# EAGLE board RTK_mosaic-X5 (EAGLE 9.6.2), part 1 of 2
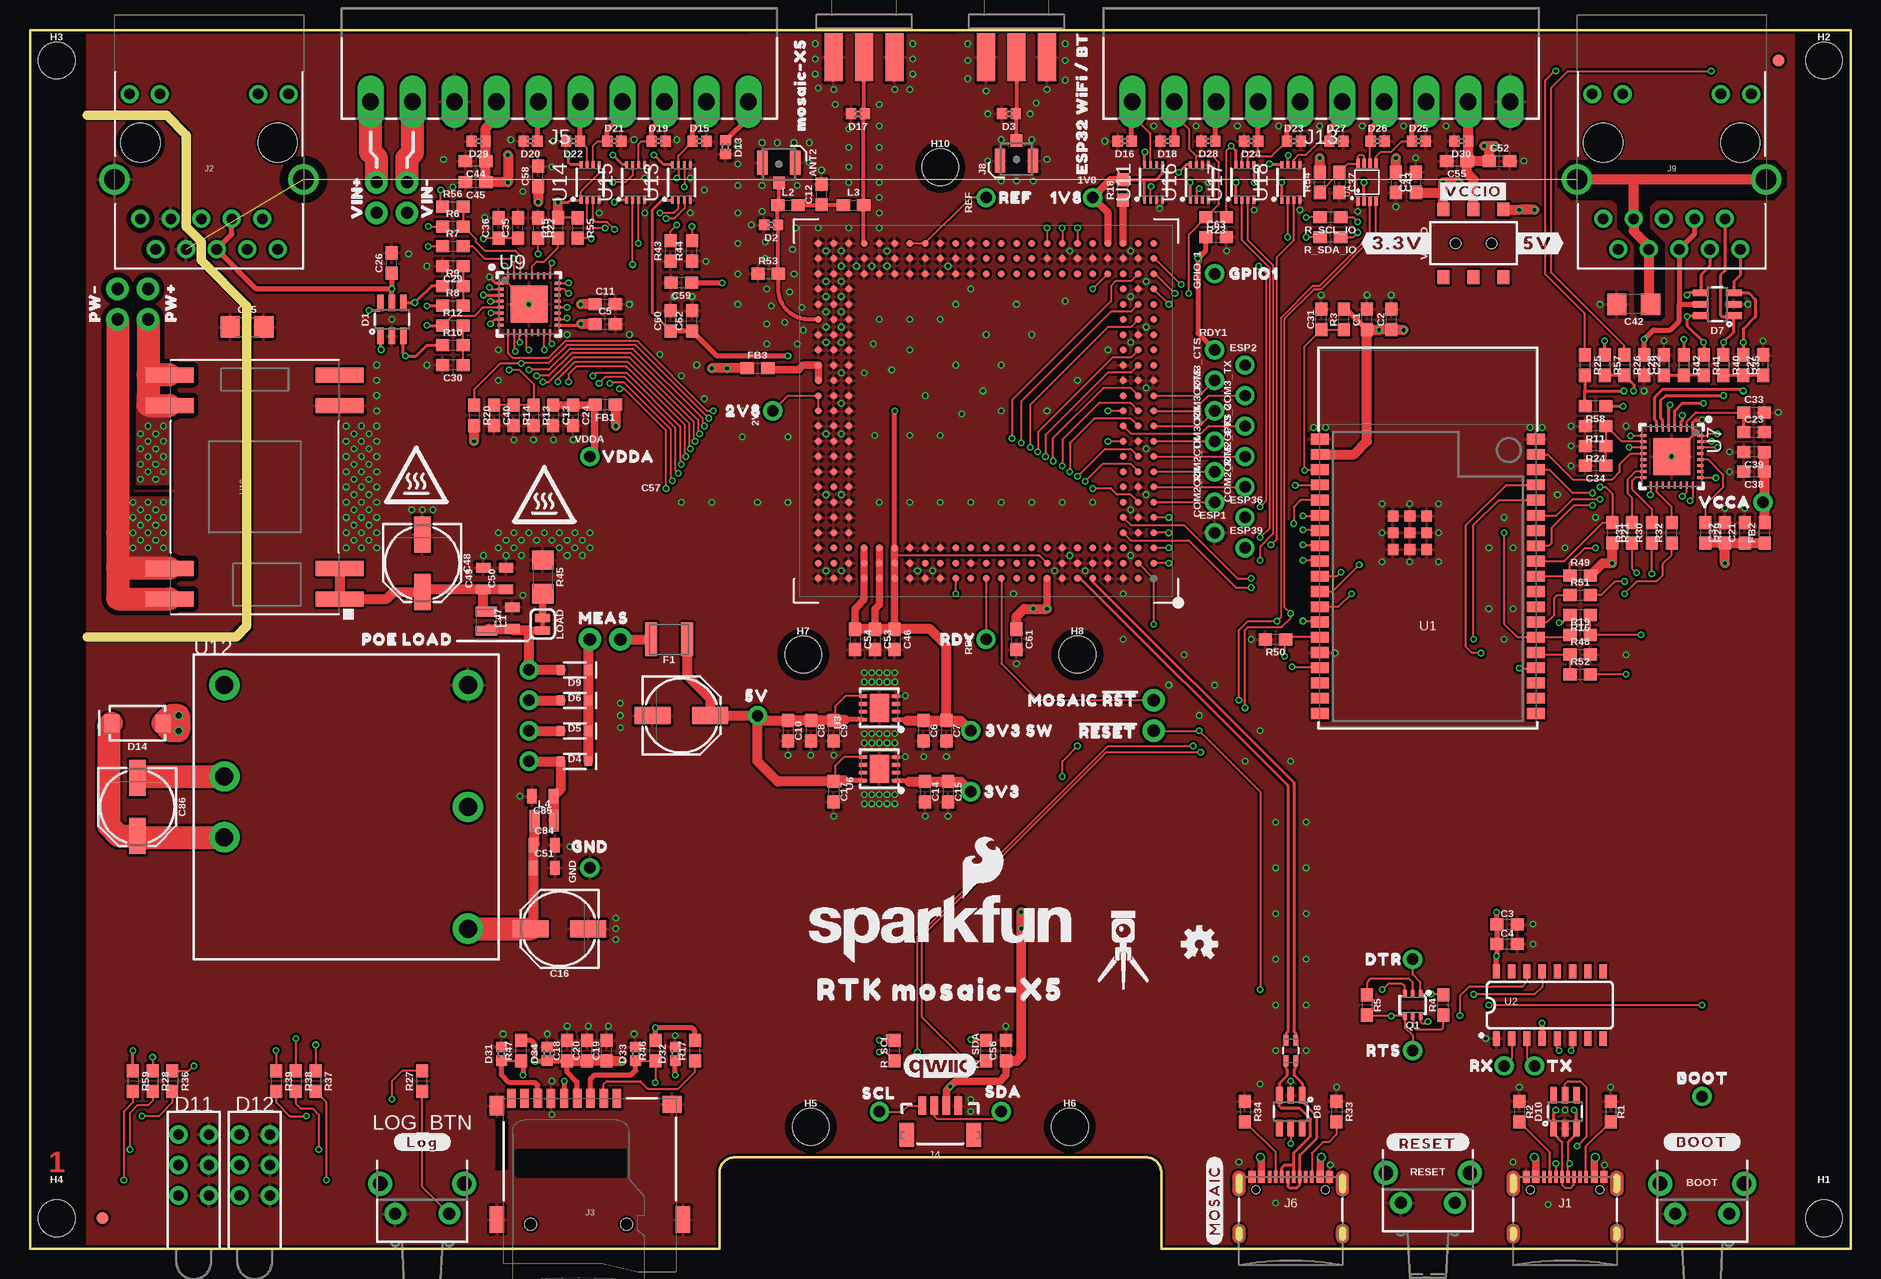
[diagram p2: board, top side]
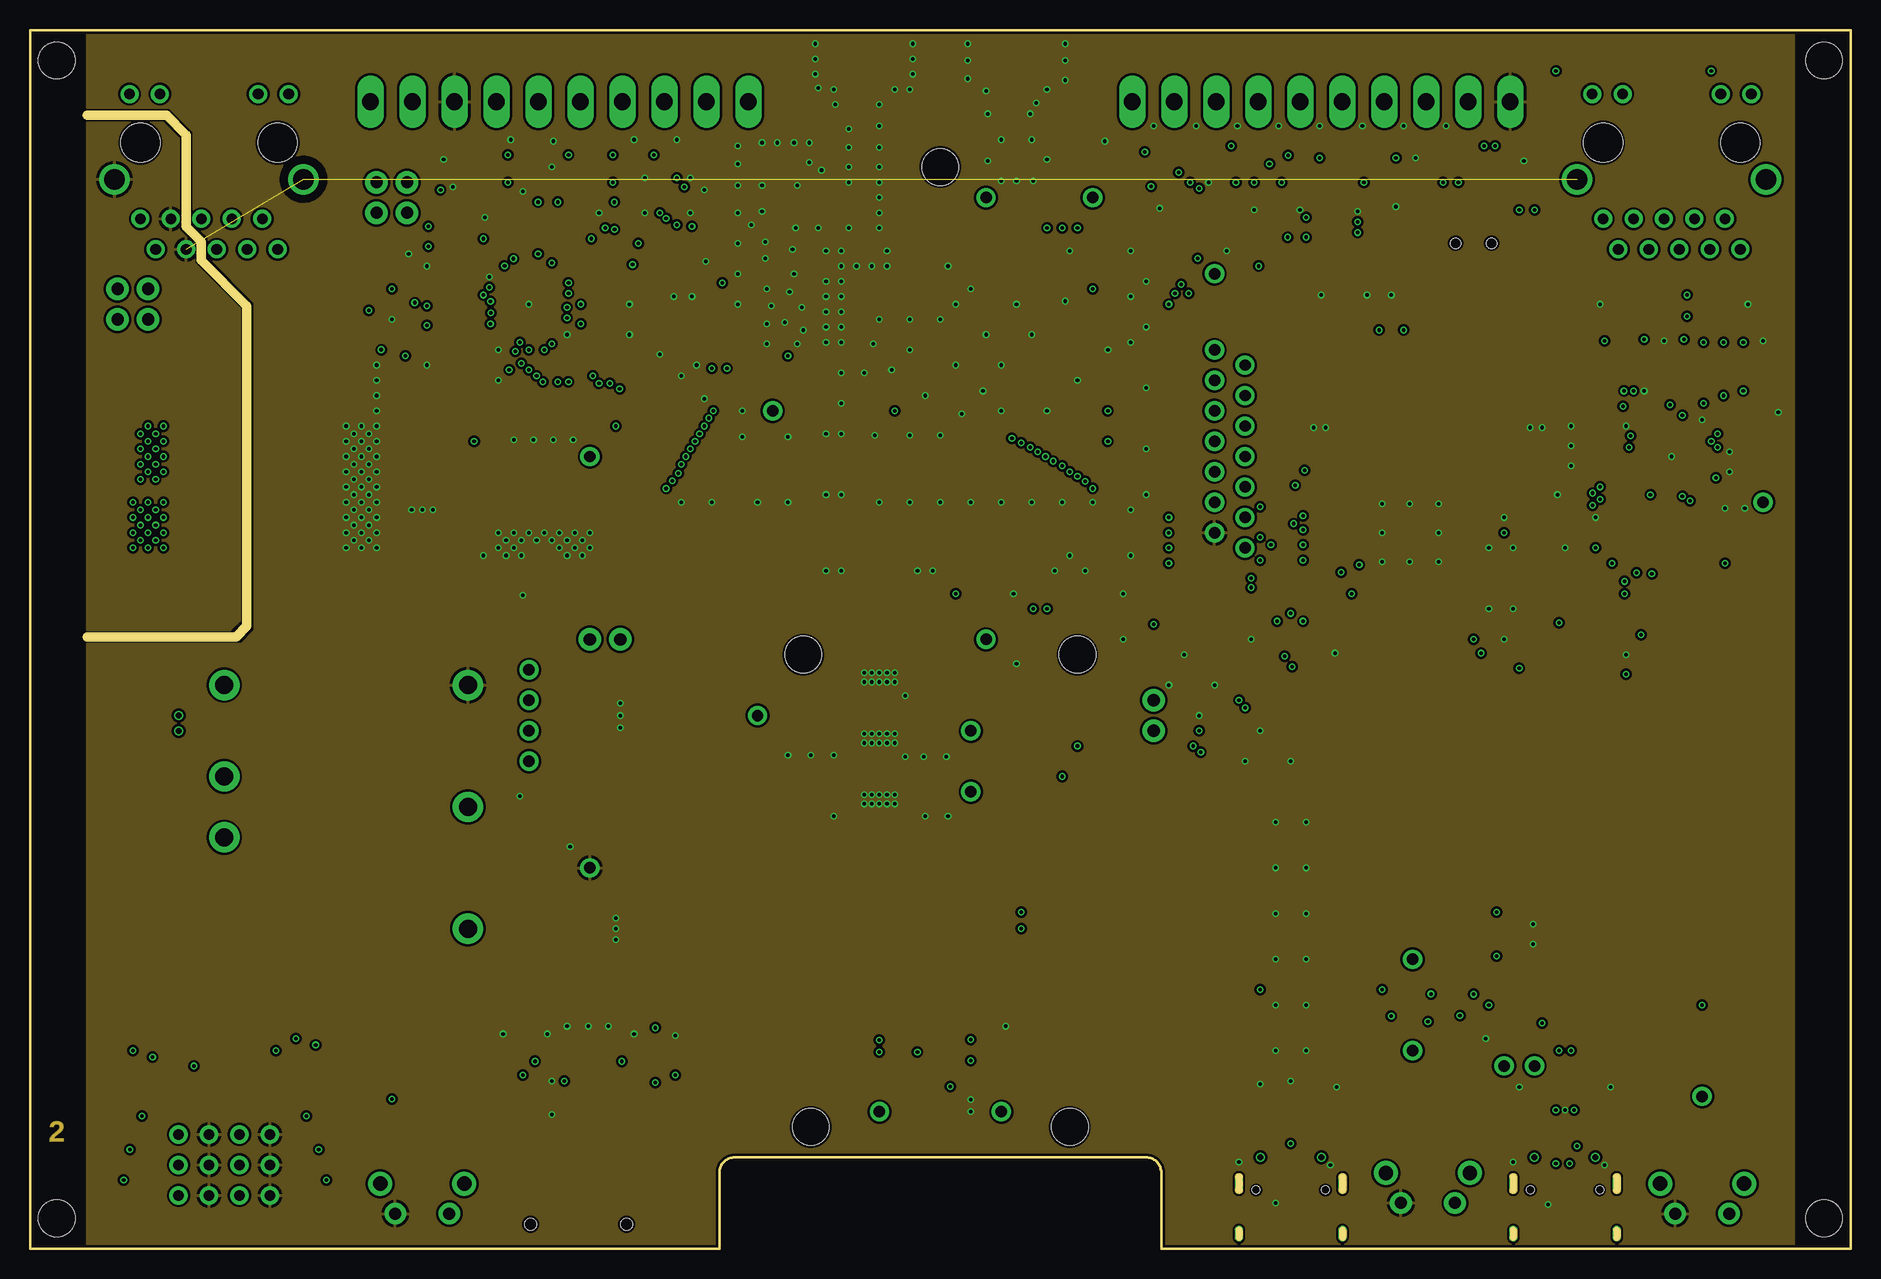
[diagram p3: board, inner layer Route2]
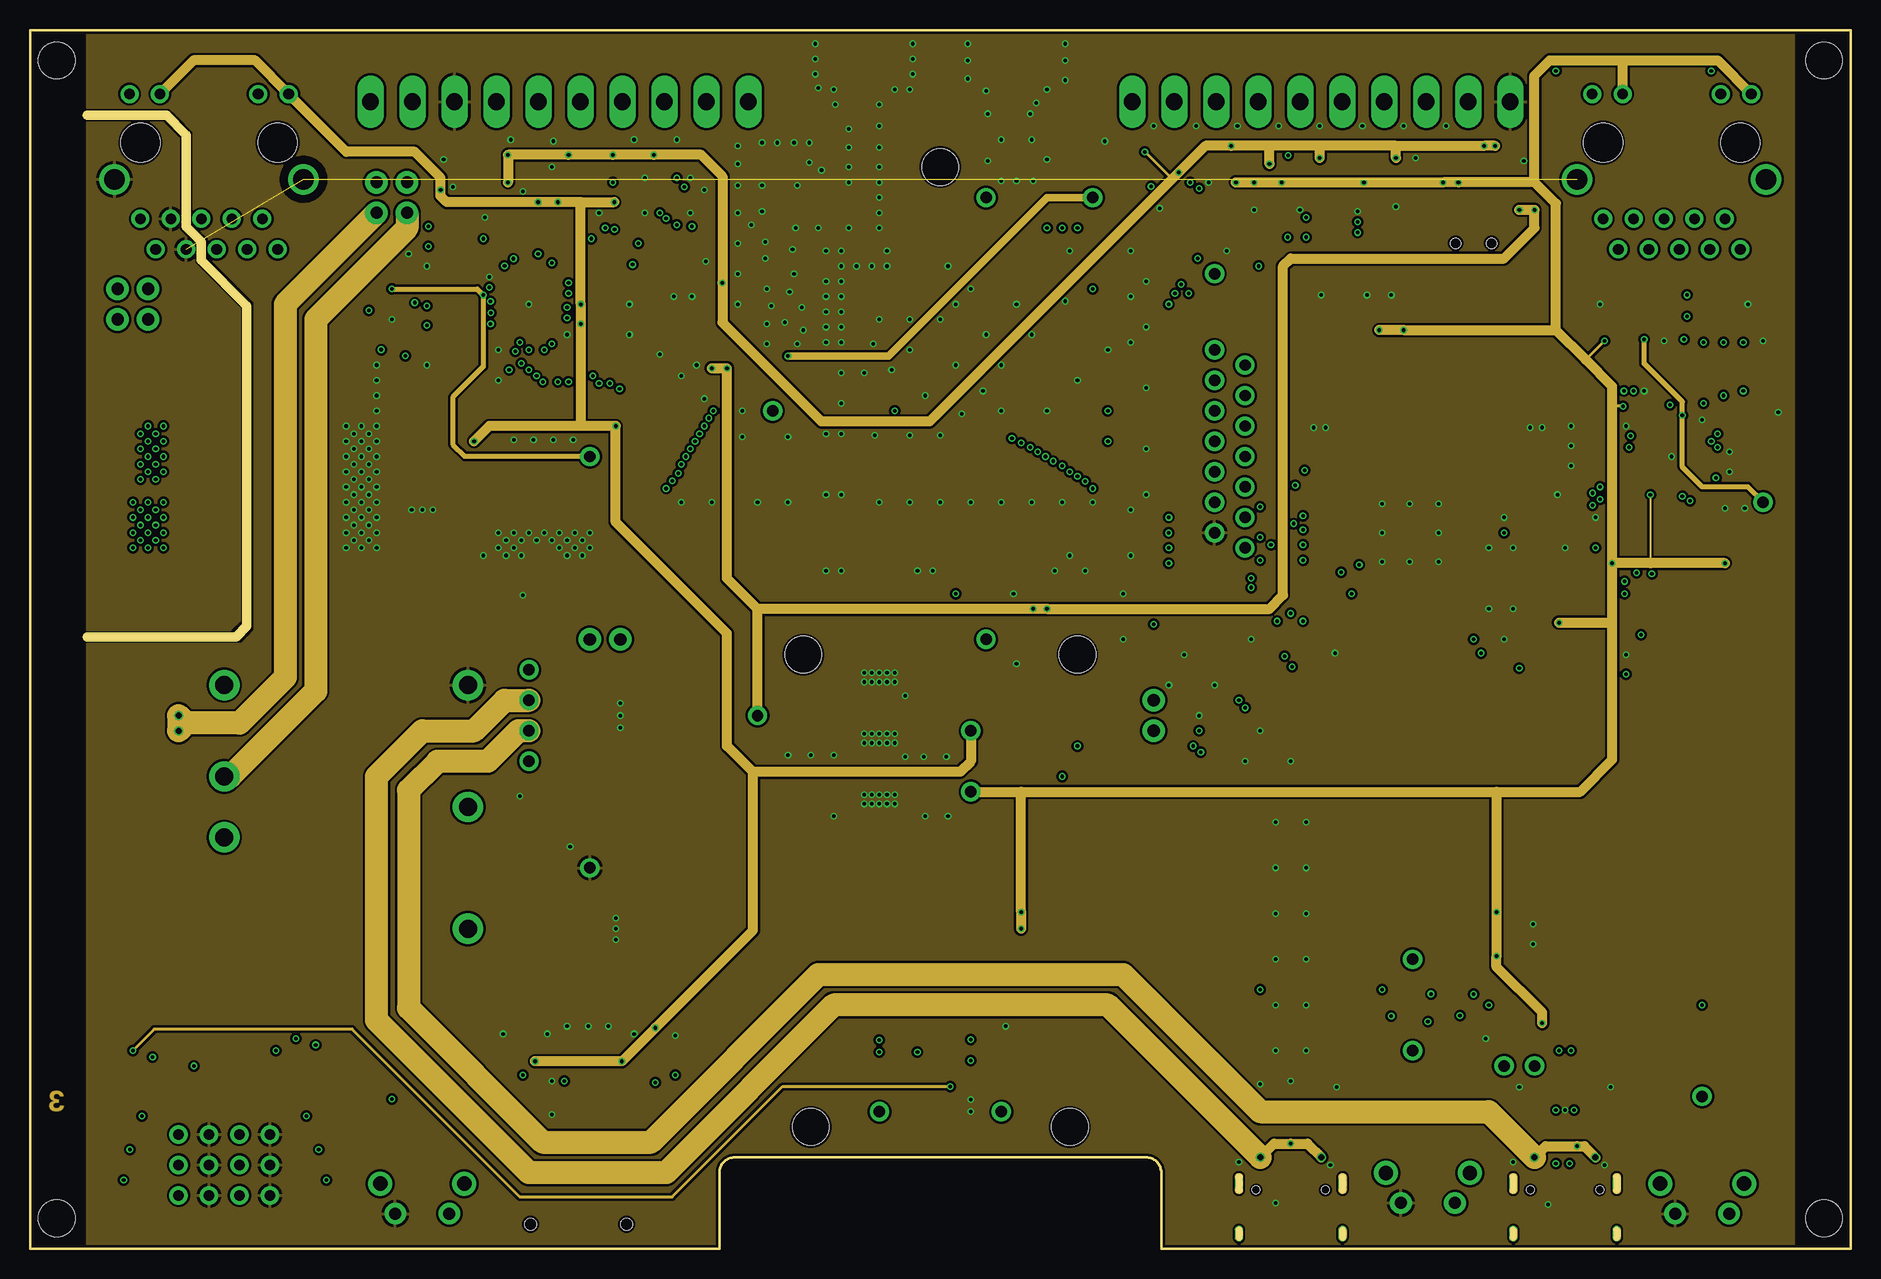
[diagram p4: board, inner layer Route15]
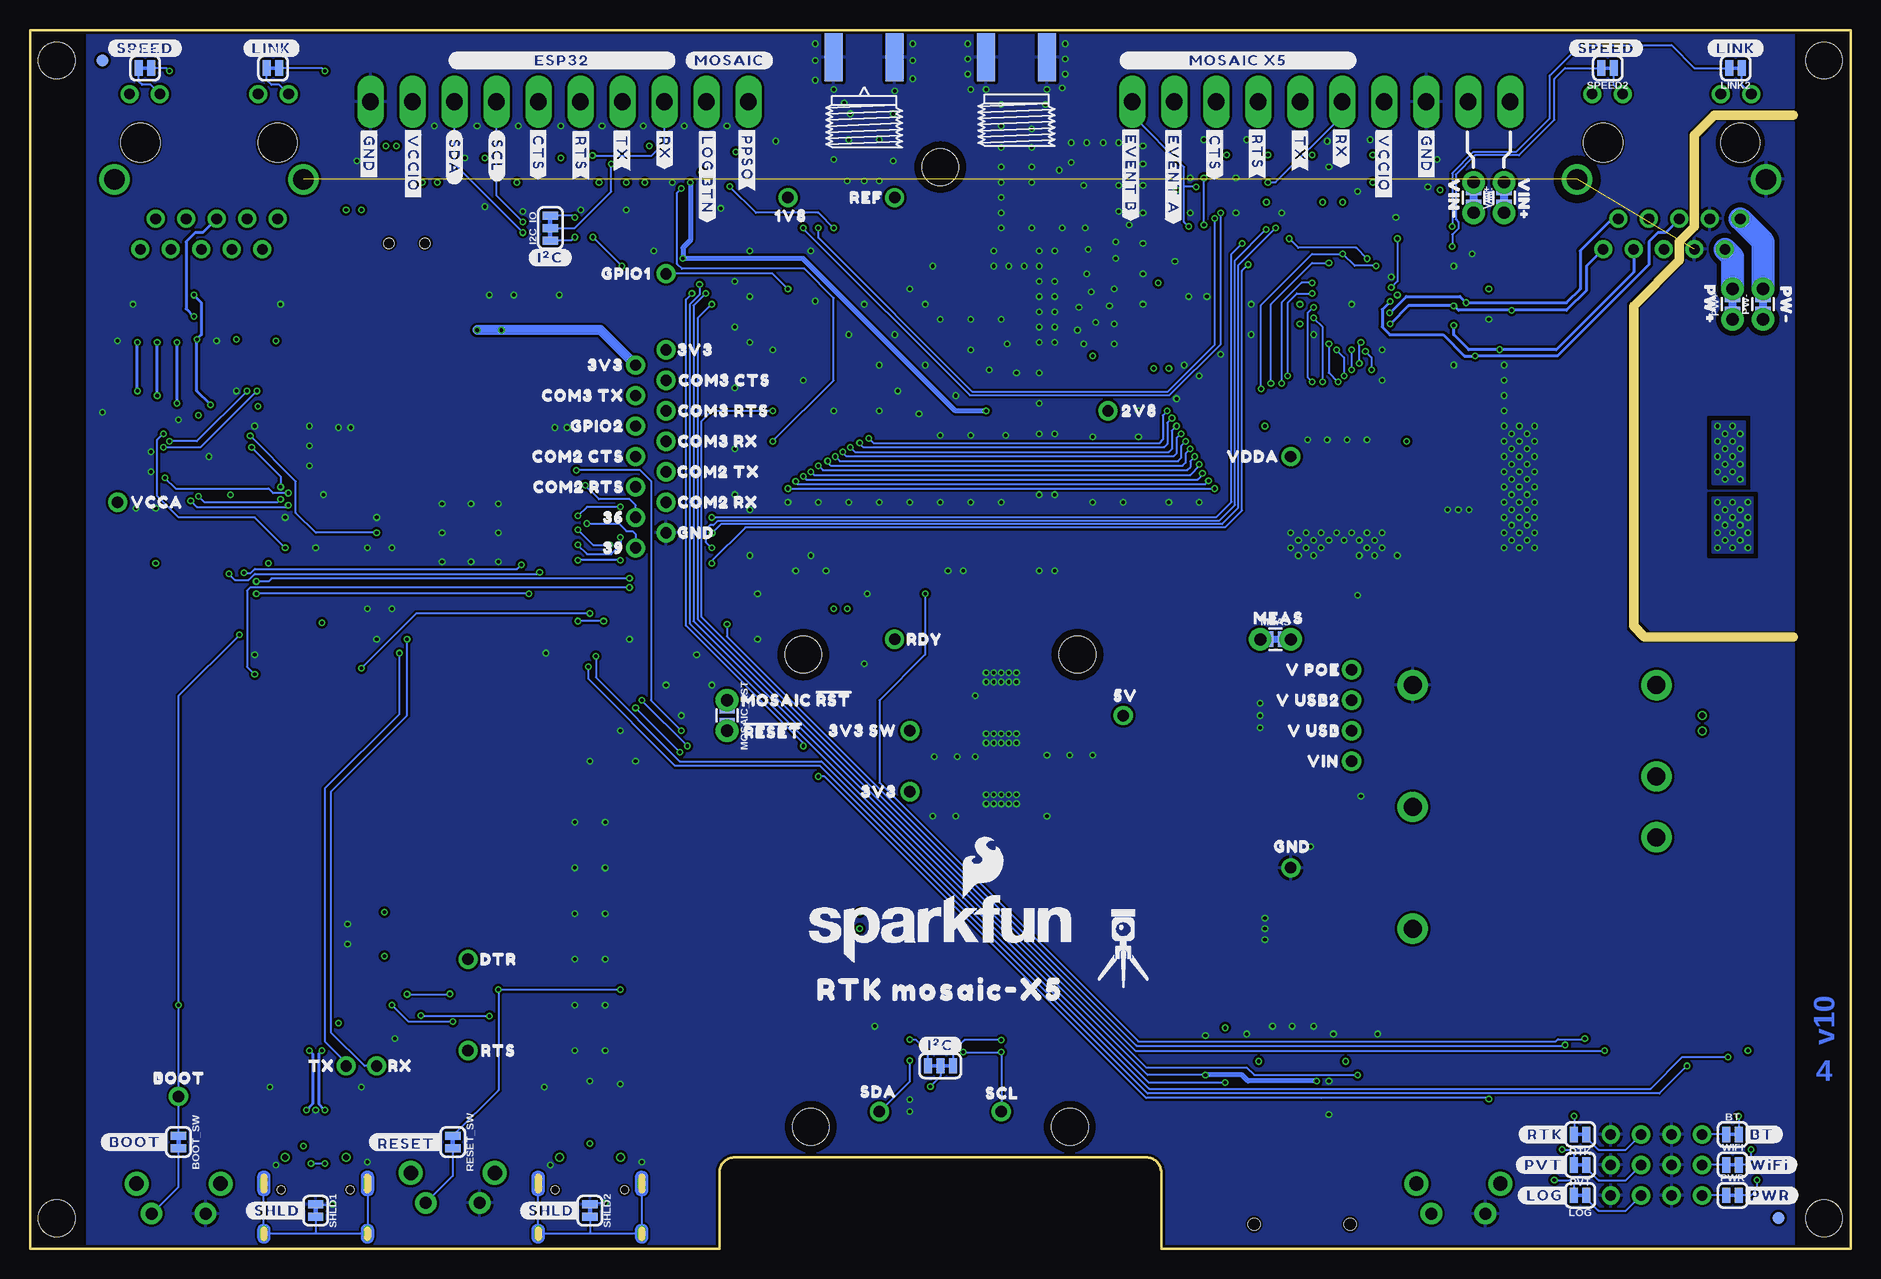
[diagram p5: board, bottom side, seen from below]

Size 151.77 x 101.6 mm. Coordinates in mm from the lower left corner, seen from the top.
Outline: 0,0 57.47,0 57.47,6.35 arc-90 58.74,7.62 93.03,7.62 arc-90 94.3,6.35 94.3,0 151.77,0 151.77,101.6 0,101.6 0,0
Copper layers (1*2*15*16): Top 0.035559375mm / dielectric 0.47751875mm / Route2 0.035559375mm / dielectric 0.47751875mm / Route15 0.035559375mm / dielectric 0.47751875mm / Bottom 0.035559375mm
Design rules "SparkFun-4-Layer-Minimum-JLCPCB": minimum track width 5mil, minimum drill 0.2mm, track to track 5mil, track to pad 5mil, pad to pad 5mil, via to via 5mil, smd to smd 5mil, copper to edge 7mil, drill to drill 7mil, minimum pad ring 5mil, minimum via ring 5mil, stop-mask expansion 2.5mil, vias tented up to drill 25mil, thermal gap 10mil
Net classes: 2 3.3V: width 0.508 mm; 3 RF_IN: width 0.35 mm, clearance 0.46 mm; 4 USB: width 0.203 mm, clearance 0.127 mm; 7 V_ZED: width 0.2 mm, clearance 0.2 mm; 8 V_RF: width 0.2 mm; 11 ZED_DIG: width 0.1 mm, clearance 0.1 mm
tKeepout: area 0,6.3 to 4.8,95.2; area 147,6.3 to 151.8,95.2
tRestrict: 3 lines
Milling: 9 lines

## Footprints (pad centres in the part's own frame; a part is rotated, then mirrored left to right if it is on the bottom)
1X01_NO_SILK = drill 0.95 pad 1.6: 1 0,0
SMA-EDGE = smd 1.5 x 4: GND@0 -2.54,0; GND@1 2.54,0; SIG 0,0 | smd 1.5 x 4 bottom: GND@2 -2.54,0; GND@3 2.54,0
U.FL_REDUCED_FOOTPRINT__NO_CREAM = smd 2 x 0.85: 1 -0.1,1.375; 2 -0.1,-1.375 | smd 1.05 x 1: FEED 1.575,0
TACTILE_SWITCH_PTH_RA_8-020 = drill 1 pad 1.8: 1 -2.25,0; 2 2.25,0 | drill 1.2 pad 2: M1 -3.5,2.5; M2 3.5,2.5
SMT-JUMPER_2_NC_TRACE_SILK = smd 0.66 x 1.27: 1 -0.521,0; 2 0.521,0
0603 = smd 1.1 x 1: 1 -0.85,0; 2 0.85,0
0603_NO_CREAM = smd 1.1 x 1: 1 -0.85,0; 2 0.85,0
PANASONIC_D = smd 3 x 1.4: + 2.4,0; - -2.4,0
1206 = smd 1.6 x 1.8: 1 -1.4,0; 2 1.4,0
0805 = smd 0.8 x 1.2: 1 -0.9,0; 2 0.9,0
SOT-23-6 = smd 0.55 x 1.35: 1 -0.95,-1.375; 2 0,-1.375; 3 0.95,-1.375; 4 0.95,1.375; 5 0,1.375; 6 -0.95,1.375
0402 = smd 0.85 x 0.9: 1 -0.58,0; 2 0.58,0
SOD-323 = smd 0.63 x 0.83: A 1.15,0; C -1.15,0
CBI_LED_T-3MM_PTH = drill 0.889 pad 1.524: ANODE_1 -1.27,9.525; ANODE_2 -1.27,6.985; ANODE_3 -1.27,4.445; CATHODE_1 1.27,9.525; CATHODE_2 1.27,6.985; CATHODE_3 1.27,4.445
SMA-DIODE = smd 1.27 x 1.47: A -2.15,0; C 2.15,0
RP-SMA-EDGE = smd 1.5 x 4: GND@0 -2.54,0; GND@1 2.54,0; SIG 0,0 | smd 1.5 x 4 bottom: GND@2 -2.54,0; GND@3 2.54,0
1210 = smd 1 x 2.8: 1 -1.5,0; 2 1.5,0
FIDUCIAL-1X2 = smd 1 x 1: 1 0,0
STAND-OFF-TIGHT = hole 3.048: 0,0
SMT-JUMPER_3_2-NC_TRACE_SILK = smd 0.66 x 1.27: 1 -1.041,0; 2 0,0; 3 1.041,0
USB-C-16P_4LAYER-PADS = smd 0.3 x 1: A5 -1.25,-0.34; A6 -0.25,-0.34; A7 0.25,-0.34; A8 1.25,-0.34; B5 1.75,-0.34; B6 0.75,-0.34; B7 -0.75,-0.34; B8 -1.75,-0.34 | smd 0.6 x 1: GND -3.225,-0.34; GND2 3.225,-0.34; VBUS1 -2.45,-0.34; VBUS2 2.45,-0.34 | drill 0.4 pad 0.6 long: SHLD1 -4.318,-0.915; SHLD2 4.318,-0.915; SHLD3 -4.318,-5.095; SHLD4 4.318,-5.095 | hole 0.65: -2.89,-1.445; 2.89,-1.445
MAGJACK-SYM_LED = drill 0.9 pad 1.5: 1 -5.715,8.89; 2 -4.445,6.35; 3 -3.175,8.89; 4 -1.905,6.35; 5 -0.635,8.89; 6 0.635,6.35; 7 1.905,8.89; 8 3.175,6.35; 9 4.445,8.89; 10 5.715,6.35; 11 -6.63,-4.06; 12 -4.09,-4.06; 13 4.09,-4.06; 14 6.63,-4.06 | drill 1.7 pad 2.4: S1 -7.875,3.05; S2 7.875,3.05 | hole 3.25: -5.715,0; 5.715,0
MICROSD-EXTERNALPIN = smd 0.7 x 1.6: 1 2.25,10.5; 2 1.15,10.5; 3 0.05,10.5; 4 -1.05,10.5; 5 -2.15,10.5; 6 -3.25,10.5; 7 -4.35,10.5; 8 -5.45,10.5; 9 -6.55,10.5 | smd 1.2 x 1.6: 10 -7.75,9.9 | smd 1.2 x 2.2: 11 -7.75,0.4; 12 7.75,0.4 | smd 1.6 x 1.4: 13 6.85,10 | hole 1: 3.05,0; -4.95,0
JST04_1MM_VERT = smd 0.6 x 1.55: 1 -1.5,0.775; 2 -0.5,0.775; 3 0.5,0.775; 4 1.5,0.775 | smd 1.2 x 2: NC1 -2.8,3.2; NC2 2.8,3.2
1X10_SCREW_TERMINAL_3.5MM = drill 1.4 pad 2.2 long: 1 -15.75,2.8; 2 -12.25,2.8; 3 -8.75,2.8; 4 -5.25,2.8; 5 -1.75,2.8; 6 1.75,2.8; 7 5.25,2.8; 8 8.75,2.8; 9 12.25,2.8; 10 15.75,2.8
U.FL_REDUCED_FOOTPRINT = smd 2 x 0.85: 1 -0.1,1.375; 2 -0.1,-1.375 | smd 1.05 x 1: FEED 1.575,0
0805-WIDE = smd 0.8 x 1.8: 1 -0.8,0; 2 0.8,0
0603_NO-CREAM = smd 1.1 x 1: 1 -0.85,0; 2 0.85,0
COMBO-JUMPER_2_NC_TRACE = smd 0.635 x 1.27: 1 -0.508,0; 2 0.508,0 | drill 1.016 pad 1.88: 3 -1.27,0; 4 1.27,0
COMBO-JUMPER_2_NO = smd 0.635 x 1.27: 1 -0.508,0; 2 0.508,0 | drill 1.016 pad 1.88: 3 -1.27,0; 4 1.27,0
SC70-6 = smd 0.3 x 0.66: 1 -0.65,-0.92; 2 0,-0.92; 3 0.65,-0.92; 4 0.65,0.92; 5 0,0.92; 6 -0.65,0.92
RFCMF1220100M4T = smd 0.9 x 0.4: A1 -0.85,0.4; A2 0.85,0.4; B1 -0.85,-0.4; B2 0.85,-0.4
ESP32-WROVER-E/IE = smd 0.9 x 1.5: 1 7.8,9; 2 6.53,9; 3 5.26,9; 4 3.99,9; 5 2.72,9; 6 1.45,9; 7 0.18,9; 8 -1.09,9; 9 -2.36,9; 10 -3.63,9; 11 -4.9,9; 12 -6.17,9; 13 -7.44,9; 14 -8.71,9; 15 -9.98,9; 16 -11.25,9; 17 -12.52,9; 18 -13.79,9; 19 -15.06,9; 20 -15.06,-9; 21 -13.79,-9; 22 -12.52,-9; 23 -11.25,-9; 24 -9.98,-9; 25 -8.71,-9; 26 -7.44,-9; 27 -6.17,-9; 28 -4.9,-9; 29 -3.63,-9; 30 -2.36,-9; 31 -1.09,-9; 32 0.18,-9; 33 1.45,-9; 34 2.72,-9; 35 3.99,-9; 36 5.26,-9; 37 6.53,-9; 38 7.8,-9 | smd 0.9 x 0.9: GND 0,1.5; GNDT1 -1.4,2.9; GNDT2 -1.4,1.5; GNDT3 -1.4,0.1; GNDT4 0,0.1; GNDT5 1.4,0.1; GNDT6 1.4,1.5; GNDT7 1.4,2.9; GNDT8 0,2.9
SO016 = smd 0.6 x 1.2: 1 -4.445,-2.8; 2 -3.175,-2.8; 3 -1.905,-2.8; 4 -0.635,-2.8; 5 0.635,-2.8; 6 1.905,-2.8; 7 3.175,-2.8; 8 4.445,-2.8; 9 4.445,2.8; 10 3.175,2.8; 11 1.905,2.8; 12 0.635,2.8; 13 -0.635,2.8; 14 -1.905,2.8; 15 -3.175,2.8; 16 -4.445,2.8
UDFN-8 = smd 0.3 x 0.65: 1 -0.975,-1.375; 2 -0.325,-1.375; 3 0.325,-1.375; 4 0.975,-1.375; 5 0.975,1.375; 6 0.325,1.375; 7 -0.325,1.375; 8 -0.975,1.375 | smd 2.35 x 1.6: EP 0,0
VSSOP_8PIN = smd 0.8 x 0.3: P1 -1.55,0.75; P2 -1.55,0.25; P3 -1.55,-0.25; P4 -1.55,-0.75; P5 1.55,-0.75; P6 1.55,-0.25; P7 1.55,0.25; P8 1.55,0.75
MLF55Q-32LD = smd 0.55 x 0.23: 1 -2.375,1.75; 2 -2.375,1.25; 3 -2.375,0.75; 4 -2.375,0.25; 5 -2.375,-0.25; 6 -2.375,-0.75; 7 -2.375,-1.25; 8 -2.375,-1.75; 17 2.375,-1.75; 18 2.375,-1.25; 19 2.375,-0.75; 20 2.375,-0.25; 21 2.375,0.25; 22 2.375,0.75; 23 2.375,1.25; 24 2.375,1.75 | smd 0.23 x 0.55: 9 -1.75,-2.375; 10 -1.25,-2.375; 11 -0.75,-2.375; 12 -0.25,-2.375; 13 0.25,-2.375; 14 0.75,-2.375; 15 1.25,-2.375; 16 1.75,-2.375; 25 1.75,2.375; 26 1.25,2.375; 27 0.75,2.375; 28 0.25,2.375; 29 -0.25,2.375; 30 -0.75,2.375; 31 -1.25,2.375; 32 -1.75,2.375 | smd 3.1 x 3.1: GND 0,0
MOSAIC_LGA = smd 0.6 x 0.6: A2 13.97,12.7; A3 13.97,11.43; A4 13.97,10.16; A5 13.97,8.89; A6 13.97,7.62; A7 13.97,6.35; A8 13.97,5.08; A9 13.97,3.81; A10 13.97,2.54; A11 13.97,1.27; A12 13.97,0; A13 13.97,-1.27; A14 13.97,-2.54; A15 13.97,-3.81; A16 13.97,-5.08; A17 13.97,-6.35; A18 13.97,-7.62; A19 13.97,-8.89; A20 13.97,-10.16; A21 13.97,-11.43; A22 13.97,-12.7; A23 13.97,-13.97; AA1 -11.43,13.97; AA2 -11.43,12.7; AA3 -11.43,11.43; AA4 -11.43,10.16; AA5 -11.43,8.89; AA6 -11.43,7.62; AA7 -11.43,6.35; AA8 -11.43,5.08; AA9 -11.43,3.81; AA10 -11.43,2.54; AA11 -11.43,1.27; AA12 -11.43,0; AA13 -11.43,-1.27; AA14 -11.43,-2.54; AA15 -11.43,-3.81; AA16 -11.43,-5.08; AA17 -11.43,-6.35; AA18 -11.43,-7.62; AA19 -11.43,-8.89; AA20 -11.43,-10.16; AA21 -11.43,-11.43; AA22 -11.43,-12.7; AA23 -11.43,-13.97; AB1 -12.7,13.97; AB2 -12.7,12.7; AB3 -12.7,11.43; AB4 -12.7,10.16; AB5 -12.7,8.89; AB6 -12.7,7.62; AB7 -12.7,6.35; AB8 -12.7,5.08; AB9 -12.7,3.81; AB10 -12.7,2.54; AB11 -12.7,1.27; AB12 -12.7,0; AB13 -12.7,-1.27; AB14 -12.7,-2.54; AB15 -12.7,-3.81; AB16 -12.7,-5.08; AB17 -12.7,-6.35; AB18 -12.7,-7.62; AB19 -12.7,-8.89; AB20 -12.7,-10.16; AB21 -12.7,-11.43; AB22 -12.7,-12.7; AB23 -12.7,-13.97; AC1 -13.97,13.97; AC2 -13.97,12.7; AC3 -13.97,11.43; AC4 -13.97,10.16; AC5 -13.97,8.89; AC6 -13.97,7.62; AC7 -13.97,6.35; AC8 -13.97,5.08; AC9 -13.97,3.81; AC10 -13.97,2.54; AC11 -13.97,1.27; AC12 -13.97,0; AC13 -13.97,-1.27; AC14 -13.97,-2.54; AC15 -13.97,-3.81; AC16 -13.97,-5.08; AC17 -13.97,-6.35; AC18 -13.97,-7.62; AC19 -13.97,-8.89; AC20 -13.97,-10.16; AC21 -13.97,-11.43; AC22 -13.97,-12.7; AC23 -13.97,-13.97; B1 12.7,13.97; B2 12.7,12.7; B3 12.7,11.43; B4 12.7,10.16; B5 12.7,8.89; B6 12.7,7.62; B7 12.7,6.35; B8 12.7,5.08; B9 12.7,3.81; B10 12.7,2.54; B11 12.7,1.27; B12 12.7,0; B13 12.7,-1.27; B14 12.7,-2.54; B15 12.7,-3.81; B16 12.7,-5.08; B17 12.7,-6.35; B18 12.7,-7.62; B19 12.7,-8.89; B20 12.7,-10.16; B21 12.7,-11.43; B22 12.7,-12.7; B23 12.7,-13.97; C1 11.43,13.97; C2 11.43,12.7; C3 11.43,11.43; C4 11.43,10.16; C5 11.43,8.89; C6 11.43,7.62; C7 11.43,6.35; C8 11.43,5.08; C9 11.43,3.81; C10 11.43,2.54; C11 11.43,1.27; C12 11.43,0; C13 11.43,-1.27; C14 11.43,-2.54; C15 11.43,-3.81; C16 11.43,-5.08; C17 11.43,-6.35; C18 11.43,-7.62; C19 11.43,-8.89; C20 11.43,-10.16; C21 11.43,-11.43; C22 11.43,-12.7; C23 11.43,-13.97; D1 10.16,13.97; D2 10.16,12.7; D3 10.16,11.43; D21 10.16,-11.43; D22 10.16,-12.7; D23 10.16,-13.97; E1 8.89,13.97; E2 8.89,12.7; E3 8.89,11.43; E21 8.89,-11.43; E22 8.89,-12.7; E23 8.89,-13.97; F1 7.62,13.97; F2 7.62,12.7; F3 7.62,11.43; F21 7.62,-11.43; F22 7.62,-12.7; F23 7.62,-13.97; G1 6.35,13.97; G2 6.35,12.7; G3 6.35,11.43; G21 6.35,-11.43; G22 6.35,-12.7; G23 6.35,-13.97; H1 5.08,13.97; H2 5.08,12.7; H3 5.08,11.43; H21 5.08,-11.43; H22 5.08,-12.7; H23 5.08,-13.97; J1 3.81,13.97; J2 3.81,12.7; J3 3.81,11.43; J21 3.81,-11.43; J22 3.81,-12.7; J23 3.81,-13.97; K1 2.54,13.97; K2 2.54,12.7; K3 2.54,11.43; K21 2.54,-11.43; K22 2.54,-12.7; K23 2.54,-13.97; L1 1.27,13.97; L2 1.27,12.7; L3 1.27,11.43; L21 1.27,-11.43; L22 1.27,-12.7; L23 1.27,-13.97; M1 0,13.97; M2 0,12.7; M3 0,11.43; M21 0,-11.43; M22 0,-12.7; M23 0,-13.97; N1 -1.27,13.97; N2 -1.27,12.7; N3 -1.27,11.43; N21 -1.27,-11.43; N22 -1.27,-12.7; N23 -1.27,-13.97; P1 -2.54,13.97; P2 -2.54,12.7; P3 -2.54,11.43; P21 -2.54,-11.43; P22 -2.54,-12.7; P23 -2.54,-13.97; R1 -3.81,13.97; R2 -3.81,12.7; R3 -3.81,11.43; R21 -3.81,-11.43; R22 -3.81,-12.7; R23 -3.81,-13.97; T1 -5.08,13.97; T2 -5.08,12.7; T3 -5.08,11.43; T21 -5.08,-11.43; T22 -5.08,-12.7; T23 -5.08,-13.97; U1 -6.35,13.97; U2 -6.35,12.7; U3 -6.35,11.43; U21 -6.35,-11.43; U22 -6.35,-12.7; U23 -6.35,-13.97; V1 -7.62,13.97; V2 -7.62,12.7; V3 -7.62,11.43; V21 -7.62,-11.43; V22 -7.62,-12.7; V23 -7.62,-13.97; W1 -8.89,13.97; W2 -8.89,12.7; W3 -8.89,11.43; W21 -8.89,-11.43; W22 -8.89,-12.7; W23 -8.89,-13.97; Y1 -10.16,13.97; Y2 -10.16,12.7; Y3 -10.16,11.43; Y21 -10.16,-11.43; Y22 -10.16,-12.7; Y23 -10.16,-13.97
DP990X = smd 1.25 x 4: 1 -9.33,-7.1; 2 -6.79,-7.1; 3 6.79,-7.1; 4 9.33,-7.1; 5 9.33,7.1; 6 6.79,7.1; 7 -6.79,7.1; 8 -9.33,7.1
VSSOP8_(SOT765-1) = smd 0.55 x 0.3: 1 -1.475,0.75; 2 -1.475,0.25; 3 -1.475,-0.25; 4 -1.475,-0.75; 5 1.475,-0.75; 6 1.475,-0.25; 7 1.475,0.25; 8 1.475,0.75
URB_YMD-15WR3 = drill 1.499 pad 2.54: 1 -10.16,10.16; 2 -10.16,2.54; 3 -10.16,-2.54; 4 10.16,-10.16; 5 10.16,0; 6 10.16,10.16
SWITCH_DPDT_SMD_AYZ0202 = smd 1 x 1.15: 1 -2.5,2.825; 2 0,2.825; 3 2.5,2.825; 4 -2.5,-2.825; 5 0,-2.825; 6 2.5,-2.825 | hole 0.85: 1.5,0; -1.5,0

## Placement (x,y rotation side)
1V8  TEST-POINTPOGO_PTH  [1X01_NO_SILK]  88.58,87.63 0 top
2V8  TEST-POINTPOGO_PTH  [1X01_NO_SILK]  61.91,69.85 90 top
3V3  TEST-POINTPOGO_PTH  [1X01_NO_SILK]  78.42,38.1 0 top
3V3_SW  TEST-POINTPOGO_PTH  [1X01_NO_SILK]  78.42,43.18 0 top
5V  TEST-POINTPOGO_PTH  [1X01_NO_SILK]  60.64,44.45 0 top
ANT1  ANTENNA-SMA-GROUNDEDEDGE_SMA  [SMA-EDGE]  69.53,99.31 0 top
ANT2  DNP  [U.FL_REDUCED_FOOTPRINT__NO_CREAM]  62.42,90.42 270 top
BOOT  MOMENTARY-SWITCH-SPST-PTH-RIGHT-ANGLE-8-020  [TACTILE_SWITCH_PTH_RA_8-020]  139.38,2.92 0 top
BOOT_SW  JUMPER-SMT_2_NC_TRACE_SILK  [SMT-JUMPER_2_NC_TRACE_SILK]  139.38,8.89 270 bottom
BT  JUMPER-SMT_2_NC_TRACE_SILK  [SMT-JUMPER_2_NC_TRACE_SILK]  9.84,9.53 0 bottom
C1  2.2uF  [0603]  111.44,77.47 90 top
C2  0.1uF  [0603]  113.47,77.47 90 top
C3  2.2uF  [0603]  123.13,27.05 0 top
C4  10nF  [0603]  123.13,25.4 0 top
C5  0.1uF  [0603]  47.94,77.09 0 top
C6  2.2uF  [0603]  74.49,43.18 270 top
C7  0.1uF  [0603]  76.39,43.18 270 top
C8  2.2uF  [0603]  65.09,43.18 270 top
C9  2.2uF  [0603]  66.99,43.18 270 top
C10  2.2uF  [0603]  63.18,43.18 270 top
C11  10uF  [0603]  47.94,78.74 0 top
C12  DNP  [0603_NO_CREAM]  65.98,87.88 90 top
C13  0.1uF  [0603]  43.62,69.47 270 top
C14  2.2uF  [0603]  74.61,38.1 270 top
C15  0.1uF  [0603]  76.52,38.1 270 top
C16  100uF  [PANASONIC_D]  44.13,26.67 180 top
C17  0.1uF  [0603]  66.99,38.1 270 top
C18  2.2uF  [0603]  44.77,16.51 90 top
C19  0.1uF  [0603]  48.07,16.51 90 top
C20  10uF  [0603]  46.42,16.51 90 top
C21  0.1uF  [0603]  142.94,59.69 90 top
C22  0.1uF  [0603]  134.56,73.66 270 top
C23  0.1uF  [0603]  143.7,68.07 0 top
C24  10uF  [0603]  45.28,69.47 270 top
C25  1nF  [1206]  18.1,76.83 0 top
C26  0.1uF  [0603]  30.16,82.17 90 top
C27  0.1uF  [0603]  144.46,73.66 90 top
C28  0.1uF  [0603]  136.21,73.66 90 top
C29  0.1uF  [0603]  35.24,81.92 180 top
C30  0.1uF  [0603]  35.24,73.66 180 top
C31  0.1uF  [0603]  107.63,77.47 90 top
C32  10uF  [0603]  141.29,59.69 90 top
C33  2.2uF  [0603]  143.7,69.72 0 top
C34  100pF  [0603]  130.49,65.28 180 top
C35  0.1uF  [0603]  40.7,85.09 90 top
C36  2.2uF  [0603]  39.05,85.09 90 top
C37  0.1uF  [0603]  109.16,88.9 270 top
C38  0.1uF  [0603]  143.7,64.77 180 top
C39  10uF  [0603]  143.7,66.42 180 top
C40  100pF  [0603]  38.67,69.47 270 top
C41  0.1uF  [0603]  115.51,88.9 90 top
C42  1nF  [1206]  133.68,78.74 180 top
C43  0.1uF  [0603]  113.86,88.9 270 top
C44  0.1uF  [0603]  37.15,90.68 180 top
C45  10uF  [0603]  37.15,88.9 180 top
C46  2.2uF  [0603]  72.07,50.8 270 top
C47  10uF  [0805]  40.2,52.58 90 top
C48  100uF  [PANASONIC_D]  32.7,57.15 270 top
C49  10uF  [0805]  37.78,55.88 90 top
C50  10uF  [0805]  39.69,55.88 90 top
C51  10uF  [0805]  42.86,31.75 0 top
C52  0.1uF  [0603]  122.49,90.68 0 top
C53  0.1uF  [0603]  70.42,50.8 270 top
C54  10uF  [0603]  68.77,50.8 270 top
C55  10uF  [0603]  118.94,90.68 180 top
C56  2.2uF  [0603]  81.34,16.51 90 top
C57  100uF  [PANASONIC_D]  54.29,44.45 0 top
C58  0.1uF  [0603]  42.35,89.41 90 top
C59  0.1uF  [0603]  54.29,80.52 180 top
C60  2.2uF  [0603]  53.4,77.34 90 top
C61  2.2uF  [0603]  82.23,50.8 270 top
C62  0.1uF  [0603]  55.18,77.34 90 top
C63  0.1uF  [0603]  98.87,84.33 0 top
C84  10uF  [0805]  42.86,33.66 0 top
C85  10uF  [0805]  42.74,37.72 180 top
C86  47UF  [PANASONIC_D]  8.95,36.83 270 top
COM2_CTS  TEST-POINTPOGO_PTH  [1X01_NO_SILK]  101.28,66.04 90 top
COM2_RTS  TEST-POINTPOGO_PTH  [1X01_NO_SILK]  101.28,63.5 90 top
COM2_RX  TEST-POINTPOGO_PTH  [1X01_NO_SILK]  98.74,62.23 90 top
COM2_TX  TEST-POINTPOGO_PTH  [1X01_NO_SILK]  98.74,64.77 90 top
COM3_CTS  TEST-POINTPOGO_PTH  [1X01_NO_SILK]  98.74,72.39 90 top
COM3_RTS  TEST-POINTPOGO_PTH  [1X01_NO_SILK]  98.74,69.85 90 top
COM3_RX  TEST-POINTPOGO_PTH  [1X01_NO_SILK]  98.74,67.31 90 top
COM3_TX  TEST-POINTPOGO_PTH  [1X01_NO_SILK]  101.28,71.12 90 top
D1  ESD Diode  [SOT-23-6]  30.16,77.47 0 top
D2  PESD0402  [0402]  61.79,85.34 180 top
D3  PESD0402  [0402]  81.6,94.61 180 top
D4  3A/10V/280mV  [SOD-323]  45.4,40.64 180 top
D5  3A/10V/280mV  [SOD-323]  45.4,43.18 180 top
D6  3A/10V/280mV  [SOD-323]  45.4,45.72 180 top
D7  ESD Diode  [SOT-23-6]  140.65,78.74 90 top
D8  ESD Diode  [SOT-23-6]  105.09,11.43 180 top
D9  3A/10V/280mV  [SOD-323]  45.4,48.26 180 top
D10  ESD Diode  [SOT-23-6]  127.95,11.43 0 top
D11  Yellow Green Red  [CBI_LED_T-3MM_PTH]  13.65,0 0 top
D12  Yellow Green Red  [CBI_LED_T-3MM_PTH]  18.73,0 0 top
D13  PESD0402  [0402]  57.98,91.82 270 top
D14  3A/40V  [SMA-DIODE]  8.95,43.81 180 top
D15  PESD0402  [0402]  55.82,92.33 0 top
D16  PESD0402  [0402]  91.25,92.33 180 top
D17  PESD0402  [0402]  69.02,94.61 180 top
D18  PESD0402  [0402]  94.81,92.33 180 top
D19  PESD0402  [0402]  52.39,92.33 0 top
D20  PESD0402  [0402]  41.72,92.33 180 top
D21  PESD0402  [0402]  48.7,92.33 0 top
D22  PESD0402  [0402]  45.28,92.33 180 top
D23  PESD0402  [0402]  105.35,92.33 0 top
D24  PESD0402  [0402]  101.79,92.33 180 top
D25  PESD0402  [0402]  115.76,92.33 0 top
D26  PESD0402  [0402]  112.33,92.33 0 top
D27  PESD0402  [0402]  108.9,92.33 0 top
D28  PESD0402  [0402]  98.23,92.33 180 top
D29  PESD0402  [0402]  37.4,92.33 180 top
D30  PESD0402  [0402]  119.32,92.33 180 top
D31  PESD0402  [0402]  39.31,16.26 90 top
D32  PESD0402  [0402]  53.78,16.26 90 top
D33  PESD0402  [0402]  50.48,16.26 90 top
D34  PESD0402  [0402]  43.12,16.26 90 top
DTR  TEST-POINTPOGO_PTH  [1X01_NO_SILK]  115.25,24.13 0 top
ESP1  TEST-POINTPOGO_PTH  [1X01_NO_SILK]  98.74,59.69 0 top
ESP2  TEST-POINTPOGO_PTH  [1X01_NO_SILK]  101.28,73.66 0 top
ESP32_RF  ANTENNA-SMA-GROUNDEDEDGE_RPSMA  [RP-SMA-EDGE]  82.23,99.31 0 top
ESP36  TEST-POINTPOGO_PTH  [1X01_NO_SILK]  101.28,60.96 0 top
ESP39  TEST-POINTPOGO_PTH  [1X01_NO_SILK]  101.28,58.42 0 top
F1  6V/2A  [1210]  53.28,50.8 180 top
FB1  470Ω  [0603]  47.94,70.36 180 top
FB2  470Ω  [0603]  144.59,59.69 90 top
FB3  470Ω  [0603]  60.64,73.41 0 top
FD1  FIDUCIAL1X2  [FIDUCIAL-1X2]  6.03,2.54 0 bottom
FD2  FIDUCIAL1X2  [FIDUCIAL-1X2]  6.03,2.54 0 top
FD3  FIDUCIAL1X2  [FIDUCIAL-1X2]  145.73,99.06 0 bottom
FD4  FIDUCIAL1X2  [FIDUCIAL-1X2]  145.73,99.06 0 top
FRAME1  FRAME-LEDGER  [CREATIVE_COMMONS]  not placed on the board
FRAME3  FRAME-LEDGERNO_FOOTPRINT  [DUMMY]  not placed on the board
GND  TEST-POINTPOGO_PTH  [1X01_NO_SILK]  46.67,31.75 90 top
GPIO_1  TEST-POINTPOGO_PTH  [1X01_NO_SILK]  98.74,81.28 90 top
GPIO_2  TEST-POINTPOGO_PTH  [1X01_NO_SILK]  101.28,68.58 90 top
H1  STAND-OFFTIGHT  [STAND-OFF-TIGHT]  149.54,2.54 0 top
H2  STAND-OFFTIGHT  [STAND-OFF-TIGHT]  149.54,99.06 0 top
H3  STAND-OFFTIGHT  [STAND-OFF-TIGHT]  2.22,99.06 0 top
H4  STAND-OFFTIGHT  [STAND-OFF-TIGHT]  2.22,2.54 0 top
H5  STAND-OFFTIGHT  [STAND-OFF-TIGHT]  65.09,10.16 0 top
H6  STAND-OFFTIGHT  [STAND-OFF-TIGHT]  86.68,10.16 0 top
H7  STAND-OFFTIGHT  [STAND-OFF-TIGHT]  64.45,49.53 0 top
H8  STAND-OFFTIGHT  [STAND-OFF-TIGHT]  87.31,49.53 0 top
H10  STAND-OFFTIGHT  [STAND-OFF-TIGHT]  75.88,90.17 0 top
I2C  JUMPER-SMT_3_2-NC_TRACE_SILK  [SMT-JUMPER_3_2-NC_TRACE_SILK]  75.88,15.24 0 bottom
I2C_IO  JUMPER-SMT_3_2-NC_TRACE_SILK  [SMT-JUMPER_3_2-NC_TRACE_SILK]  108.39,85.09 90 bottom
J1  [USB-C-16P_4LAYER-PADS]  127.95,6.35 0 top
J2  MAGJACK-POE  [MAGJACK-SYM_LED]  14.92,92.2 180 top
J3  MICRO-SD-PUSH-PUSH-EXT-PIN  [MICROSD-EXTERNALPIN]  46.67,2.03 0 top
J4  Vertical Qwiic Connector  [JST04_1MM_VERT]  75.88,12.7 180 top
J5  [1X10_SCREW_TERMINAL_3.5MM]  44.13,98.42 180 top
J6  [USB-C-16P_4LAYER-PADS]  105.09,6.35 0 top
J8  [U.FL_REDUCED_FOOTPRINT]  82.23,90.81 90 top
J9  MAGJACK-POE  [MAGJACK-SYM_LED]  136.84,92.2 180 top
J13  [1X10_SCREW_TERMINAL_3.5MM]  107.63,98.42 180 top
L1  2.2uH  [0805-WIDE]  38.04,52.32 270 top
L2  DNP  [0603_NO-CREAM]  63.18,87 0 top
L3  DNP  [0603_NO-CREAM]  68.64,87 0 top
L4  2.2uH  [0805-WIDE]  42.86,35.69 0 top
LINK  JUMPER-SMT_2_NC_TRACE_SILK  [SMT-JUMPER_2_NC_TRACE_SILK]  131.51,98.42 0 bottom
LINK2  JUMPER-SMT_2_NC_TRACE_SILK  [SMT-JUMPER_2_NC_TRACE_SILK]  9.59,98.42 180 bottom
LOAD  JUMPER-SMT_2_NC_TRACE_SILK  [SMT-JUMPER_2_NC_TRACE_SILK]  42.74,52.07 270 top
LOG  JUMPER-SMT_2_NC_TRACE_SILK  [SMT-JUMPER_2_NC_TRACE_SILK]  22.54,4.45 180 bottom
LOG_BTN  MOMENTARY-SWITCH-SPST-PTH-RIGHT-ANGLE-8-020  [TACTILE_SWITCH_PTH_RA_8-020]  32.7,2.92 0 top
LOGO1  SPECIAL_INSTRUCTIONS-ORDERING  [ORDERING_INSTRUCTIONS]  not placed on the board
LOGO2  QWIIC_LOGO_6MM  [QWIIC_6MM]  75.88,15.24 0 top
LOGO4  OSHW-LOGOS  [OSHW-LOGO-S]  97.47,25.4 0 top
LOGO5  SFE_LOGO_NAME.2_INCH  [SFE_LOGO_NAME_.2]  75.88,26.67 0 top
LOGO6  SFE_LOGO_FLAME.2_INCH  [SFE_LOGO_FLAME_.2]  79.44,31.75 0 top
LOGO7  SFE_LOGO_NAME.2_INCH  [SFE_LOGO_NAME_.2]  75.88,26.67 0 bottom
LOGO8  SFE_LOGO_FLAME.2_INCH  [SFE_LOGO_FLAME_.2]  72.33,31.75 0 bottom
MEAS  JUMPER-COMBO_2_NC_TRACE  [COMBO-JUMPER_2_NC_TRACE]  47.94,50.8 0 bottom
MOSAIC_RST  JUMPER-COMBO_2_NO  [COMBO-JUMPER_2_NO]  93.66,44.45 270 bottom
PVT  JUMPER-SMT_2_NC_TRACE_SILK  [SMT-JUMPER_2_NC_TRACE_SILK]  22.54,6.99 180 bottom
PW+  JUMPER-COMBO_2_NC_TRACE  [COMBO-JUMPER_2_NC_TRACE]  9.84,78.74 90 bottom
PW-  JUMPER-COMBO_2_NC_TRACE  [COMBO-JUMPER_2_NC_TRACE]  7.3,78.74 90 bottom
PWR  JUMPER-SMT_2_NC_TRACE_SILK  [SMT-JUMPER_2_NC_TRACE_SILK]  9.84,4.45 0 bottom
Q1  [SC70-6]  115.25,20.32 180 top
R1  5.1k  [0603]  131.76,11.43 270 top
R2  5.1k  [0603]  124.14,11.43 270 top
R3  10k  [0603]  109.54,77.47 90 top
R4  10k  [0603]  117.79,20.32 90 top
R5  10k  [0603]  111.44,20.32 270 top
R6  1k  [0603]  35.24,85.22 0 top
R7  1k  [0603]  35.24,83.57 0 top
R8  49.9  [0603]  35.24,78.61 0 top
R9  49.9  [0603]  35.24,80.26 0 top
R10  49.9  [0603]  35.24,75.31 0 top
R11  13k  [0603]  130.49,68.58 180 top
R12  49.9  [0603]  35.24,76.96 0 top
R13  13k  [0603]  41.97,69.47 270 top
R14  13k  [0603]  40.32,69.47 270 top
R15  10k  [0603]  44.01,85.09 90 top
R16  10k  [0603]  129.22,52.83 180 top
R17  10k  [0603]  55.44,16.51 90 top
R18  10k  [0603]  91.12,88.27 90 top
R19  1k  [0603]  129.22,51.18 0 top
R20  4.7k  [0603]  37.02,69.47 270 top
R21  4.7k  [0603]  131.89,59.69 270 top
R22  10k  [0603]  42.35,85.09 270 top
R23  10k  [0603]  98.87,85.98 180 top
R24  13k  [0603]  130.49,66.93 180 top
R25  1k  [0603]  129.6,73.66 270 top
R26  1k  [0603]  132.91,73.66 270 top
R27  1k  [0603]  32.7,13.97 90 top
R28  470  [0603]  10.22,13.97 270 top
R29  10k  [0603]  139.64,59.69 270 top
R30  33  [0603]  135.19,59.69 90 top
R31  33  [0603]  133.54,59.69 90 top
R32  33  [0603]  136.84,59.69 90 top
R33  5.1k  [0603]  108.9,11.43 270 top
R34  5.1k  [0603]  101.28,11.43 270 top
R35  49.9  [0603]  142.81,73.66 270 top
R36  470  [0603]  11.87,13.97 270 top
R37  470  [0603]  23.81,13.97 270 top
R38  470  [0603]  22.16,13.97 270 top
R39  470  [0603]  20.51,13.97 270 top
R40  49.9  [0603]  141.16,73.66 270 top
R41  49.9  [0603]  139.51,73.66 270 top
R42  49.9  [0603]  137.86,73.66 270 top
R43  10k  [0603]  53.4,83.19 90 top
R44  10k  [0603]  55.18,83.19 90 top
R45  49.9 1/2W  [1206]  42.74,56.01 270 top
R46  10k  [0603]  52.13,16.51 90 top
R47  10k  [0603]  40.96,16.51 90 top
R48  10k  [0603]  129.22,49.53 0 top
R49  10k  [0603]  129.22,56.13 0 top
R50  10k  [0603]  103.82,50.8 180 top
R51  0  [0603]  129.22,54.48 0 top
R52  0  [0603]  129.22,47.88 0 top
R53  0  [0603]  61.53,81.28 0 top
R54  200k  [0603]  107.51,88.9 90 top
R55  4.7k  [0603]  45.66,85.09 270 top
R56  4.7k  [0603]  35.24,86.87 0 top
R57  4.7k  [0603]  131.25,73.66 270 top
R58  4.7k  [0603]  130.49,70.23 180 top
R59  470  [0603]  8.57,13.97 270 top
R_SCL  2.2k  [0603]  72.07,16.51 90 top
R_SCL_IO  2.2k  [0603]  108.39,85.98 180 top
R_SDA  2.2k  [0603]  79.69,16.51 90 top
R_SDA_IO  2.2k  [0603]  108.39,84.33 180 top
RDY  TEST-POINTPOGO_PTH  [1X01_NO_SILK]  79.69,50.8 90 top
RDY1  TEST-POINTPOGO_PTH  [1X01_NO_SILK]  98.74,74.93 0 top
REF  TEST-POINTPOGO_PTH  [1X01_NO_SILK]  79.69,87.63 90 top
RESET  MOMENTARY-SWITCH-SPST-PTH-RIGHT-ANGLE-8-020  [TACTILE_SWITCH_PTH_RA_8-020]  116.52,3.81 0 top
RESET_SW  JUMPER-SMT_2_NC_TRACE_SILK  [SMT-JUMPER_2_NC_TRACE_SILK]  116.52,8.89 270 bottom
RTK  JUMPER-SMT_2_NC_TRACE_SILK  [SMT-JUMPER_2_NC_TRACE_SILK]  22.54,9.53 180 bottom
RTS  TEST-POINTPOGO_PTH  [1X01_NO_SILK]  115.25,16.51 0 top
RX  TEST-POINTPOGO_PTH  [1X01_NO_SILK]  122.87,15.24 0 top
SCL2  TEST-POINTPOGO_PTH  [1X01_NO_SILK]  70.8,11.43 0 top
SDA2  TEST-POINTPOGO_PTH  [1X01_NO_SILK]  80.96,11.43 0 top
SHLD1  JUMPER-SMT_2_NC_TRACE_SILK  [SMT-JUMPER_2_NC_TRACE_SILK]  127.95,3.17 270 bottom
SHLD2  JUMPER-SMT_2_NC_TRACE_SILK  [SMT-JUMPER_2_NC_TRACE_SILK]  105.09,3.17 270 bottom
SPEED  JUMPER-SMT_2_NC_TRACE_SILK  [SMT-JUMPER_2_NC_TRACE_SILK]  142.18,98.42 0 bottom
SPEED2  JUMPER-SMT_2_NC_TRACE_SILK  [SMT-JUMPER_2_NC_TRACE_SILK]  20.26,98.42 180 bottom
T1  TRANSFORMER0508  [RFCMF1220100M4T]  105.09,16.51 270 top
TP_BOOT  TEST-POINTPOGO_PTH  [1X01_NO_SILK]  139.38,12.7 0 top
TX  TEST-POINTPOGO_PTH  [1X01_NO_SILK]  125.41,15.24 0 top
U1  ESP32-WROVER-IE  [ESP32-WROVER-E/IE]  116.52,59.69 90 top
U2  CH340C  [SO016]  126.68,20.32 0 top
U3  AP7361C-33FGEUDFN-8  [UDFN-8]  70.8,45.09 90 top
U4  [VSSOP_8PIN]  111.44,88.9 90 top
U6  AP7361C-33FGEUDFN-8  [UDFN-8]  70.8,40.01 90 top
U7  KSZ8041NLI  [MLF55Q-32LD]  136.84,66.04 270 top
U8  MOSAIC-X5X5  [MOSAIC_LGA]  79.69,69.85 270 top
U9  KSZ8041NLI  [MLF55Q-32LD]  41.59,78.74 0 top
U10  POE_PSU-DP990X  [DP990X]  18.73,63.5 90 top
U11  [VSSOP8_(SOT765-1)]  93.66,88.9 90 top
U12  URB2405YMD  [URB_YMD-15WR3]  26.35,36.83 0 top
U13  [VSSOP8_(SOT765-1)]  54.29,88.9 90 top
U14  [VSSOP8_(SOT765-1)]  46.67,88.9 90 top
U15  [VSSOP8_(SOT765-1)]  50.48,88.9 90 top
U16  [VSSOP8_(SOT765-1)]  97.47,88.9 90 top
U17  [VSSOP8_(SOT765-1)]  101.28,88.9 90 top
U18  [VSSOP8_(SOT765-1)]  105.09,88.9 90 top
U$2  [MOSAIC#X50]  64.2,97.03 90 top
U$3  [#SHLD#0]  105.73,3.17 0 bottom
U$4  [#RESET#0]  89.85,43.18 0 top
U$5  [PW#0]  5.4,76.58 90 top
U$6  [PW#1]  11.75,76.58 90 top
U$7  [##RESET##5]  117.28,8.89 0 bottom
U$8  [#I�C#0]  108.39,82.61 0 bottom
U$9  [MOSAIC_#RST#6]  93.03,45.85 0 top
U$10  [#LINK#1]  131.64,100.08 0 bottom
U$11  [#LOG#4]  23.3,4.45 0 bottom
U$12  [#PVT#2]  23.3,6.99 0 bottom
U$13  [#RTK#3]  23.3,9.53 0 bottom
U$14  [#BT#2]  9.08,9.53 0 bottom
U$15  [#BOOT#6]  140.14,8.89 0 bottom
U$16  [#_______________MOSAIC_X5_______________#8]  41.21,99.06 0 bottom
U$17  [#RX#2]  42.48,90.17 270 bottom
U$18  [#TX#3]  45.91,89.92 270 bottom
U$19  [#RTS#4]  49.47,89.28 270 bottom
U$20  [#CTS#5]  53.02,89.15 270 bottom
U$21  [ESP32_WIFI_#_BT0]  87.69,102.11 90 top
U$22  [#EVENT_A#6]  56.45,85.47 270 bottom
U$23  [#EVENT_B#7]  60.01,85.72 270 bottom
U$24  [VCCA0]  141.29,62.23 0 top
U$25  [#GND#0]  35.37,89.03 270 bottom
U$26  [#VCCIO#1]  38.93,87.38 270 bottom
U$27  [#VCCIO#1]  119.82,87.38 270 bottom
U$28  [#GND#0]  123.51,89.03 270 bottom
U$29  [#RTS#4]  105.85,89.15 270 bottom
U$30  [#CTS#5]  109.41,89.15 270 bottom
U$31  [#RX#2]  98.87,90.04 270 bottom
U$32  [#TX#3]  102.43,89.92 270 bottom
U$33  [#PPSO#11]  92.01,88.27 270 bottom
U$34  [#LOG_BTN#33]  95.31,85.6 270 bottom
U$35  [#SCL#10]  112.84,89.03 270 bottom
U$36  [#SDA#9]  116.4,88.77 270 bottom
U$37  [#MOSAIC#8]  89.85,99.06 0 bottom
U$38  [#___________________ESP32___________________#34]  97.98,99.06 0 bottom
U$39  [#3#3V#6]  117.03,83.82 0 top
U$40  [#5V#0]  127.83,83.82 0 top
U$41  [2V8220]  61.66,69.85 0 top
U$42  [2V8220]  57.09,69.85 0 bottom
U$43  [BOOT2]  142.3,14.22 0 top
U$44  [BOOT2]  136.46,14.22 0 bottom
U$45  [#SHLD#0]  128.59,3.17 0 bottom
U$46  [#I�C#0]  75.88,16.95 0 bottom
U$47  [COM2_CTS219]  101.54,66.04 0 bottom
U$48  [COM2_RTS219]  101.54,63.5 0 bottom
U$49  [COM2_RX219]  90.36,62.23 0 bottom
U$54  [COM2_TX219]  90.23,64.77 0 bottom
U$55  [RTS2231]  112.84,16.51 0 top
U$56  [DTR2232]  112.84,24.13 0 top
U$57  [COM3_CTS18]  89.34,72.39 0 bottom
U$58  [COM3_RTS18]  89.47,69.85 0 bottom
U$59  [3V3_SW25]  86.04,43.18 0 top
U$60  [3V325]  83.25,38.1 0 top
U$61  [5V25]  62.29,46.1 0 top
U$62  [MEAS2]  50.61,52.58 0 top
U$63  [VIN#0]  27.24,87.5 270 bottom
U$64  [COM3_RX219]  90.36,67.31 0 bottom
U$65  [COM3_TX18]  101.54,71.12 0 bottom
U$66  [GPIO17]  104.84,81.28 0 top
U$67  [GPIO17]  99.25,81.28 0 bottom
U$68  [GPIO218]  101.54,68.58 0 bottom
U$69  [RTK_MOSAIC#X50]  75.88,21.59 0 top
U$70  [VIN#0]  27.24,87.63 90 top
U$71  [VIN#1]  33.08,87.5 270 bottom
U$72  [VIN#1]  33.08,87.63 90 top
U$73  [MOSAIC_#RST#6]  82.61,45.85 0 bottom
U$74  [#RESET#0]  89.85,43.18 0 bottom
U$75  [RDY5]  79.57,50.8 0 top
U$76  [RTS2231]  112.71,16.51 0 bottom
U$77  [DTR2232]  112.71,24.13 0 bottom
U$78  [RDY5]  74.99,50.8 0 bottom
U$79  [REF219]  84.26,87.63 0 top
U$80  [REF219]  79.95,87.63 0 bottom
U$81  [V_POE0]  41.85,48.26 0 bottom
U$82  [V_USB3]  41.85,43.18 0 bottom
U$83  [V_USB24]  41.85,45.72 0 bottom
U$84  [MEAS2]  44.89,52.58 0 bottom
U$85  [VIN1]  41.97,40.64 0 bottom
U$86  [5V25]  58.74,46.1 0 bottom
U$87  [3V325]  78.8,38.1 0 bottom
U$88  [3V3_SW25]  78.8,43.18 0 bottom
U$89  [RX0]  122.75,15.24 0 top
U$90  [RX0]  119.19,15.24 0 bottom
U$91  [SCL3]  72.83,12.95 0 top
U$92  [SCL3]  68.64,12.95 0 bottom
U$93  [SDA4]  83.38,13.08 0 top
U$94  [SDA4]  78.8,13.08 0 bottom
U$95  [TX1]  129.35,15.24 0 top
U$96  [TX1]  125.67,15.24 0 bottom
U$97  [VDDA220]  52.77,66.04 0 top
U$98  [VDDA220]  46.93,66.04 0 bottom
U$99  [RTK_MOSAIC#X50]  75.88,21.59 0 bottom
U$100  [#VCCIO#1]  123.38,88.14 0 top
U$101  [1V80]  88.46,87.63 0 top
U$102  [1V80]  86.3,86.11 0 bottom
U$103  [#PWR#0]  9.08,4.45 0 bottom
U$104  [#WIFI#1]  9.08,6.99 0 bottom
U$105  [360]  104.71,60.96 0 bottom
U$106  [39361]  104.71,58.42 0 bottom
U$107  [VCCA0]  141.16,62.23 0 bottom
U$108  [GND39362]  98.49,59.69 0 bottom
U$109  [3V339362]  105.98,73.66 0 bottom
U$110  [3V339362]  98.49,74.93 0 bottom
U$113  [PW#0]  5.4,80.9 270 bottom
U$114  [PW#1]  11.75,81.03 270 bottom
U$116  [#_LOG_#5]  32.7,8.89 0 top
U$117  [#_#RESET#_#0]  116.52,8.89 0 top
U$118  [#_BOOT_#1]  139.38,8.89 0 top
U$119  [#MOSAIC#8]  98.74,7.62 90 top
U$120  [#LINK#1]  9.59,100.08 0 bottom
U$121  [#SPEED#0]  20.38,100.08 0 bottom
U$122  [#SPEED#0]  142.18,100.08 0 bottom
U$135  [GND12]  46.55,33.53 0 bottom
U$136  [POE_LOAD0]  31.43,50.8 0 top
U$143  [GND12]  46.67,33.53 0 top
U$146  [HIGH_TEMP_WARNING]  42.86,62.23 0 top
U$147  [HIGH_TEMP_WARNING]  32.19,63.88 0 top
U$152  [RTK5#SVG0]  91.12,24.89 0 top
U$153  [RTK5#SVG0]  60.64,25.02 0 bottom
VCCA  TEST-POINTPOGO_PTH  [1X01_NO_SILK]  144.46,62.23 0 top
VCCIO  [SWITCH_DPDT_SMD_AYZ0202]  120.33,83.82 0 top
VDDA  TEST-POINTPOGO_PTH  [1X01_NO_SILK]  46.67,66.04 0 top
VIN  TEST-POINTPOGO_PTH  [1X01_NO_SILK]  41.59,40.64 0 top
VIN+  JUMPER-COMBO_2_NC_TRACE  [COMBO-JUMPER_2_NC_TRACE]  28.89,87.63 90 bottom
VIN-  JUMPER-COMBO_2_NC_TRACE  [COMBO-JUMPER_2_NC_TRACE]  31.43,87.63 270 bottom
VPOE  TEST-POINTPOGO_PTH  [1X01_NO_SILK]  41.59,48.26 0 top
VUSB  TEST-POINTPOGO_PTH  [1X01_NO_SILK]  41.59,43.18 0 top
VUSB2  TEST-POINTPOGO_PTH  [1X01_NO_SILK]  41.59,45.72 0 top
WIFI  JUMPER-SMT_2_NC_TRACE_SILK  [SMT-JUMPER_2_NC_TRACE_SILK]  9.84,6.99 0 bottom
